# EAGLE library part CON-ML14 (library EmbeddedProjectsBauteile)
HARTING Wannenstecker 2x7 polig
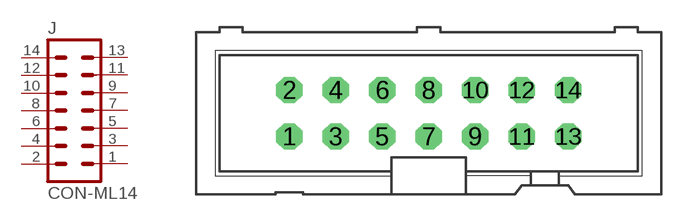
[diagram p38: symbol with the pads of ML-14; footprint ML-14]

Designator prefix J

## CON-ML14 (EP: 400506)  [ML-14]
1  1  pas
2  2  pas
3  3  pas
4  4  pas
5  5  pas
6  6  pas
7  7  pas
8  8  pas
9  9  pas
10  10  pas
11  11  pas
12  12  pas
13  13  pas
14  14  pas

## Footprint ML-14 (pad centres in mm)
drill 0.914 octagon: 1 -7.62,-1.27; 2 -7.62,1.27; 3 -5.08,-1.27; 4 -5.08,1.27; 5 -2.54,-1.27; 6 -2.54,1.27; 7 0,-1.27; 8 0,1.27; 9 2.54,-1.27; 10 2.54,1.27; 11 5.08,-1.27; 12 5.08,1.27; 13 7.62,-1.27; 14 7.62,1.27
